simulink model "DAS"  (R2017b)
settings: Solver=FixedStepDiscrete  StartTime=0.0  StopTime=10.0  FixedStep=0.01  RelTol=1e-3  EnableMultiTasking=on
undefined symbols (not defined in the file): CcDAS_ACModeCurtLim_A, CcDAS_ACModeCurtTiLim_ms, CcDAS_BMSOperationConfirmTi_ms, CcDAS_CellMaxTempLim1_C, CcDAS_CellMaxTempLim2_C, CcDAS_CellMaxTempLim3_C, CcDAS_CellMaxTempLim4_C, CcDAS_CellMinTempHiLim_C, CcDAS_CellMinTempLowLim_C, CcDAS_CellMinTempMidLim_C, CcDAS_CellTempDiffLim_C, CcDAS_DCModeCurtTiLim_ms, CcDAS_HVSafetyNVMStoreTi_ms, CcDAS_OCVSOCDiffLim1_numb, CcDAS_OCVSOCDiffLim2_numb, CcDAS_PackCurrLim_A, CcDAS_SOCHighLim_numb, CcDAS_SOCLowerLim_numb, CcDAS_SOHLowerLim_numb, CcDAS_SOHLowerLimSale_numb, DAS_MIN2MS_NUMB, DAS_RUNTIME100_MS, DAS_RUNTIME10_MS, DAS_STATSTIMEMAX_MIN, DAS_STATSTIMEMIN_MIN, DAS_STATSTIMESMAX_NUMB, DAS_STATSTIMESMIN_NUMB, DAS_TIMESONE_NUMB, Enum_CTCCtrCtlConnMode
libraries: AIWAYS_Powertrain_BMS_lib x268
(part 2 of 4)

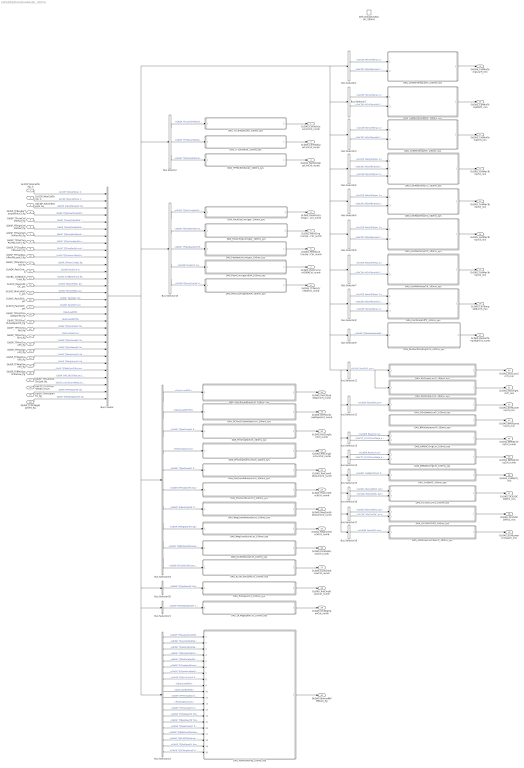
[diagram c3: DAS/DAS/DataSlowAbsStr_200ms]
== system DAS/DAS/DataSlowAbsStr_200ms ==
  GcCDP_MinCellTemp_C : Inport
  GcCDP_MaxCellTemp_C : Inport  Port=2
  GbCDP_AllCellTempVld_flg : Inport  Port=3
  GbISP_TFBusbarTempHiFltLv3_flg : Inport  Port=4
  GbISP_TFLowCellVoltSaf_flg : Inport  Port=5
  GbISP_TFHighCellVoltSaf_flg : Inport  Port=6
  GbISP_TFPackVoltHiAlrmFlt_flg : Inport  Port=7
  GbISP_TFDisChrgPwrFltLevel3_flg : Inport  Port=8
  GbISP_TFChrgPwrFltLevel3_flg : Inport  Port=9
  GbISP_TFFeedbackPwrFltLevel3_flg : Inport  Port=10
  GbISP_TFPackCrntSaf_flg : Inport  Port=11
  GcHDP_PackCrnt_A : Inport  Port=12
  GaCBC_CellBalCtlCmd_flg : Inport  Port=13
  GcSOC_MaxCellSOC_pct : Inport  Port=14
  GcSOC_MinCellSOC_pct : Inport  Port=15
  GcSOC_PackSOC_pct : Inport  Port=16
  GcSOH_PackSOH_pct : Inport  Port=17
  GbISP_TFPosCtlLoadOpenFlt_flg : Inport  Port=18
  GbISP_TFDCPosCtlLoadOpenFlt_flg : Inport  Port=19
  GbISP_TFPreChrgFail_flg : Inport  Port=20
  GbISP_TFPreChrgShrt_flg : Inport  Port=21
  GbISP_TFPosCloseFlt_flg : Inport  Port=22
  GbISP_TFPosOpenFlt_flg : Inport  Port=23
  GbISP_TFNegCloseFlt_flg : Inport  Port=24
  GbISP_TFNegOpenFlt_flg : Inport  Port=25
  GbISP_TFBMUSpyStTooLow_flg : Inport  Port=26
  GbISP_TFKL30CStTooLow_flg : Inport  Port=27
  GeCTC_CtrCtlConnMode_enum : Inport  Port=28
  GbISP_TFPreOpenFlt_flg : Inport  Port=29
  GbISP_TFDCNegOpenFlt_flg : Inport  Port=30
  DAS_DataSlowAbsStr_200ms : TriggerPort  TriggerType=function-call  VariantControl=(inherit)
  Bus Creator : BusCreator  Inputs=30
  Bus Selector : BusSelector  OutputSignals=GbISP_TFLowCellVoltSaf_flg,GbISP_TFHighCellVoltSaf_flg,GbISP_TFPackVoltHiAlrmFlt_flg
  Bus Selector1 : BusSelector  OutputSignals=GcCDP_MinCellTemp_C,GbCDP_AllCellTempVld_flg
  Bus Selector10 : BusSelector  OutputSignals=GbISP_TFDisChrgPwrFltLevel3_flg,GbISP_TFChrgPwrFltLevel3_flg,GbISP_TFFeedbackPwrFltLevel3_flg,GcHDP_PackCrnt_A,GbISP_TFPackCrntSaf_flg
  Bus Selector11 : BusSelector  OutputSignals=GcSOC_PackSOC_pct
  Bus Selector12 : BusSelector  OutputSignals=GcSOH_PackSOH_pct
  Bus Selector13 : BusSelector  OutputSignals=GcHDP_PackCrnt_A,GeCTC_CtrCtlConnMode_enum
  Bus Selector14 : BusSelector  OutputSignals=GcHDP_PackCrnt_A,GeCTC_CtrCtlConnMode_enum
  Bus Selector15 : BusSelector  OutputSignals=GaCBC_CellBalCtlCmd_flg
  Bus Selector16 : BusSelector  OutputSignals=GcSOC_MaxCellSOC_pct,GcSOC_MinCellSOC_pct
  Bus Selector17 : BusSelector  OutputSignals=GcSOC_MaxCellSOC_pct,GcSOC_MinCellSOC_pct
  Bus Selector18 : BusSelector  OutputSignals=OpenLoadPOS,OpenLoadDCPOS,GbISP_TFPreChrgFail_flg,PreChrgOverCurt,GbISP_TFPosCloseFlt_flg,GbISP_TFPosOpenFlt_flg,GbISP_TFNegCloseFlt_flg,GbISP_TFNegOpenFlt_flg,GbISP_TFBMUSpyStTooLow_flg,GbISP_TFKL30CStTooLow_flg
  Bus Selector19 : BusSelector  OutputSignals=GcSOH_PackSOH_pct
  Bus Selector2 : BusSelector  OutputSignals=GcCDP_MinCellTemp_C,GbCDP_AllCellTempVld_flg
  Bus Selector20 : BusSelector  OutputSignals=GbISP_TFPreOpenFlt_flg
  Bus Selector21 : BusSelector  OutputSignals=GbISP_TFDCNegOpenFlt_flg
  Bus Selector22 : BusSelector  OutputSignals=GbISP_TFBusbarTempHiFltLv3_flg,GbISP_TFLowCellVoltSaf_flg,GbISP_TFHighCellVoltSaf_flg,GbISP_TFPackVoltHiAlrmFlt_flg,GbISP_TFDisChrgPwrFltLevel3_flg,GbISP_TFChrgPwrFltLevel3_flg,GbISP_TFFeedbackPwrFltLevel3_flg,GbISP_TFPackCrntSaf_flg,OpenLoadPOS,OpenLoadDCPOS,GbISP_TFPreChrgFail_flg,PreChrgOverCurt,GbISP_TFPosCloseFlt_flg,GbISP_TFPosOpenFlt_flg,GbISP_TFNegOpenFlt_flg,GbISP_TFNegCloseFlt_flg,GbISP_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
  Bus Selector3 : BusSelector  OutputSignals=GcCDP_MinCellTemp_C,GbCDP_AllCellTempVld_flg
  Bus Selector4 : BusSelector  OutputSignals=GcCDP_MaxCellTemp_C,GbCDP_AllCellTempVld_flg,GcCDP_MinCellTemp_C
  Bus Selector5 : BusSelector  OutputSignals=GcCDP_MaxCellTemp_C,GbCDP_AllCellTempVld_flg
  Bus Selector6 : BusSelector  OutputSignals=GcCDP_MaxCellTemp_C,GbCDP_AllCellTempVld_flg
  Bus Selector7 : BusSelector  OutputSignals=GcCDP_MaxCellTemp_C,GbCDP_AllCellTempVld_flg
  Bus Selector8 : BusSelector  OutputSignals=GcCDP_MaxCellTemp_C,GbCDP_AllCellTempVld_flg,GcCDP_MinCellTemp_C
  Bus Selector9 : BusSelector  OutputSignals=GbISP_TFBusbarTempHiFltLv3_flg
  DAS_BMSACChrgCnt_100ms_sys : Subsystem  TreatAsAtomicUnit=on
  DAS_BMSDCChrgCnt_100ms_sys : Subsystem  TreatAsAtomicUnit=on
  DAS_BMSOperationTi_100ms_sys : Subsystem  TreatAsAtomicUnit=on
  DAS_BusbarTempHighCnt_100ms_sys : Subsystem  TreatAsAtomicUnit=on
  DAS_CellBalTi_100ms_sys : Subsystem  TreatAsAtomicUnit=on
  DAS_CellMaxTempTi1_100ms_sys : Subsystem  TreatAsAtomicUnit=on
  DAS_CellMaxTempTi2_100ms_sys : Subsystem  TreatAsAtomicUnit=on
  DAS_CellMaxTempTi3_100ms_sys : Subsystem  TreatAsAtomicUnit=on
  DAS_CellMaxTempTi4_100ms_sys : Subsystem  TreatAsAtomicUnit=on
  DAS_CellMinTempHiTi_100ms_sys : Subsystem  TreatAsAtomicUnit=on
  DAS_CellMinTempLowTi_100ms_sys : Subsystem  TreatAsAtomicUnit=on
  DAS_CellMinTempMidTi_100ms_sys : Subsystem  TreatAsAtomicUnit=on
  DAS_CellTempDiffTi_100ms_sys : Subsystem  TreatAsAtomicUnit=on
  DAS_DCNegOpenCnt_100ms_sys : Subsystem  TreatAsAtomicUnit=on
  DAS_DCPosCtlLoadOpenCnt_100ms_sys : Subsystem  TreatAsAtomicUnit=on
  DAS_FeedbackCurrUppr_100ms_sys : Subsystem  TreatAsAtomicUnit=on
  DAS_KL30CVoltLowCnt_100ms_sys : Subsystem  TreatAsAtomicUnit=on
  DAS_KL30VoltLowCnt_100ms_sys : Subsystem  TreatAsAtomicUnit=on
  DAS_NVMStoreFlg_100ms_sys : Subsystem  TreatAsAtomicUnit=on
  DAS_NegContAdhesionCnt_100ms_sys : Subsystem  TreatAsAtomicUnit=on
  DAS_NegContStuckCnt_100ms_sys : Subsystem  TreatAsAtomicUnit=on
  DAS_OCVSOCDiff1_100ms_sys : Subsystem  TreatAsAtomicUnit=on
  DAS_OCVSOCDiff2_100ms_sys : Subsystem  TreatAsAtomicUnit=on
  DAS_PACKCurrUppr600A_100ms_sys : Subsystem  TreatAsAtomicUnit=on
  DAS_PackChrgCurrUppr_100ms_sys : Subsystem  TreatAsAtomicUnit=on
  DAS_PackCurrUppr500A_100ms_sys : Subsystem  TreatAsAtomicUnit=on
  DAS_PackDisCurrUppr_100ms_sys : Subsystem  TreatAsAtomicUnit=on
  DAS_PosContAdhesionCnt_100ms_sys : Subsystem  TreatAsAtomicUnit=on
  DAS_PosContStuckCnt_100ms_sys : Subsystem  TreatAsAtomicUnit=on
  DAS_PosCtlLoadOpenCnt_100ms_sys : Subsystem  TreatAsAtomicUnit=on
  DAS_PreChrgFailCnt_100ms_sys : Subsystem  TreatAsAtomicUnit=on
  DAS_PreChrgOverCurtCnt_100ms_sys : Subsystem  TreatAsAtomicUnit=on
  DAS_PreOpenCnt_100ms_sys : Subsystem  TreatAsAtomicUnit=on
  DAS_SOCHighLimTi_100ms_sys : Subsystem  TreatAsAtomicUnit=on
  DAS_SOCUpprLimTi_100ms_sys : Subsystem  TreatAsAtomicUnit=on
  DAS_SOHLowerLimSaleTi_100ms_sys : Subsystem  TreatAsAtomicUnit=on
  DAS_SOHLowerLimTi_100ms_sys : Subsystem  TreatAsAtomicUnit=on
  DAS_TFCellVoltHi_100ms_sys : Subsystem  TreatAsAtomicUnit=on
  DAS_TFCellVoltLowr_100ms_sys : Subsystem  TreatAsAtomicUnit=on
  DAS_TFPACKVoltLowr_100ms_sys : Subsystem  TreatAsAtomicUnit=on
  GcDAS_CellVoltLowrLimCnt_numb : Outport
  GcDAS_CellVoltUpprLimCnt_numb : Outport  Port=2
  GcDAS_BattVoltUpprLimCnt_numb : Outport  Port=3
  GcDAS_PackDisCurrUpprLimCnt_numb : Outport  Port=4
  GcDAS_PackChrgCurrUpprLimCnt_numb : Outport  Port=5
  GcDAS_FeedbackCurrUpprLimCnt_numb : Outport  Port=6
  GcDAS_PackCurrLim500ACnt_numb : Outport  Port=7
  GcDAS_TFPackCrntSafCnt_numb : Outport  Port=8
  GcDAS_CellMinTempLowTi_min : Outport  Port=9
  GcDAS_CellMinTempMidTi_min : Outport  Port=10
  GcDAS_CellMinTempHiTi_min : Outport  Port=11
  GcDAS_CellMaxTempTi1_min : Outport  Port=12
  GcDAS_CellMaxTempTi2_min : Outport  Port=13
  GcDAS_CellMaxTempTi3_min : Outport  Port=14
  GcDAS_CellMaxTempTi4_min : Outport  Port=15
  GcDAS_CellTempDiffLimTi_min : Outport  Port=16
  GcDAS_BusbarTempHighCnt_numb : Outport  Port=17
  GcDAS_PosCtlLoadOpenCnt_numb : Outport  Port=18
  GcDAS_DCPosCtlLoadOpenCnt_numb : Outport  Port=19
  GcDAS_PreChrgFailCnt_numb : Outport  Port=20
  GcDAS_PreChrgOvrCurrCnt_numb : Outport  Port=21
  GcDAS_PosContAdhesionCnt_numb : Outport  Port=22
  GcDAS_PosContStuckCnt_numb : Outport  Port=23
  GcDAS_NegContAdhesionCnt_numb : Outport  Port=24
  GcDAS_NegContStuckCnt_numb : Outport  Port=25
  GcDAS_KL30VoltLowCnt_numb : Outport  Port=26
  GcDAS_KL30CVoltLowCnt_numb : Outport  Port=27
  GcDAS_PreChrgOpenCnt_numb : Outport  Port=28
  GcDAS_DCNegOpenCnt_numb : Outport  Port=29
  GcDAS_SOCLowLimTi_min : Outport  Port=30
  GcDAS_SOCHighLimTi_min : Outport  Port=31
  GcDAS_SOHLowerLimTi_min : Outport  Port=32
  GcDAS_BMSOperationTi_min : Outport  Port=33
  GcDAS_BMSACChrgCnt_numb : Outport  Port=34
  GcDAS_BMSDCChrgCnt_numb : Outport  Port=35
  GcDAS_CellBalTi_min : Outport  Port=36
  GcDAS_OCVSOCDiffTi1_min : Outport  Port=37
  GcDAS_OCVSOCDiffTi2_min : Outport  Port=38
  GcDAS_SOHLowerLimSaleTi_min : Outport  Port=39
  GbDAS_NormalNVMStore_flg : Outport  Port=40
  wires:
  GcCDP_MinCellTemp_C/1 -> Bus Creator/1  "GcCDP_MinCellTemp_C"
  GcCDP_MaxCellTemp_C/1 -> Bus Creator/2  "GcCDP_MaxCellTemp_C"
  GbCDP_AllCellTempVld_flg/1 -> Bus Creator/3  "GbCDP_AllCellTempVld_flg"
  GbISP_TFBusbarTempHiFltLv3_flg/1 -> Bus Creator/4  "GbISP_TFBusbarTempHiFltLv3_flg"
  GbISP_TFLowCellVoltSaf_flg/1 -> Bus Creator/5  "GbISP_TFLowCellVoltSaf_flg"
  GbISP_TFHighCellVoltSaf_flg/1 -> Bus Creator/6  "GbISP_TFHighCellVoltSaf_flg"
  GbISP_TFPackVoltHiAlrmFlt_flg/1 -> Bus Creator/7  "GbISP_TFPackVoltHiAlrmFlt_flg"
  GbISP_TFDisChrgPwrFltLevel3_flg/1 -> Bus Creator/8  "GbISP_TFDisChrgPwrFltLevel3_flg"
  GbISP_TFChrgPwrFltLevel3_flg/1 -> Bus Creator/9  "GbISP_TFChrgPwrFltLevel3_flg"
  GbISP_TFFeedbackPwrFltLevel3_flg/1 -> Bus Creator/10  "GbISP_TFFeedbackPwrFltLevel3_flg"
  GbISP_TFPackCrntSaf_flg/1 -> Bus Creator/11  "GbISP_TFPackCrntSaf_flg"
  GcHDP_PackCrnt_A/1 -> Bus Creator/12  "GcHDP_PackCrnt_A"
  GaCBC_CellBalCtlCmd_flg/1 -> Bus Creator/13  "GaCBC_CellBalCtlCmd_flg"
  GcSOC_MaxCellSOC_pct/1 -> Bus Creator/14  "GcSOC_MaxCellSOC_pct"
  GcSOC_MinCellSOC_pct/1 -> Bus Creator/15  "GcSOC_MinCellSOC_pct"
  GcSOC_PackSOC_pct/1 -> Bus Creator/16  "GcSOC_PackSOC_pct"
  GcSOH_PackSOH_pct/1 -> Bus Creator/17  "GcSOH_PackSOH_pct"
  GbISP_TFPosCtlLoadOpenFlt_flg/1 -> Bus Creator/18  "OpenLoadPOS"
  GbISP_TFDCPosCtlLoadOpenFlt_flg/1 -> Bus Creator/19  "OpenLoadDCPOS"
  GbISP_TFPreChrgFail_flg/1 -> Bus Creator/20  "GbISP_TFPreChrgFail_flg"
  GbISP_TFPreChrgShrt_flg/1 -> Bus Creator/21  "PreChrgOverCurt"
  GbISP_TFPosCloseFlt_flg/1 -> Bus Creator/22  "GbISP_TFPosCloseFlt_flg"
  GbISP_TFPosOpenFlt_flg/1 -> Bus Creator/23  "GbISP_TFPosOpenFlt_flg"
  GbISP_TFNegCloseFlt_flg/1 -> Bus Creator/24  "GbISP_TFNegCloseFlt_flg"
  GbISP_TFNegOpenFlt_flg/1 -> Bus Creator/25  "GbISP_TFNegOpenFlt_flg"
  GbISP_TFBMUSpyStTooLow_flg/1 -> Bus Creator/26  "GbISP_TFBMUSpyStTooLow_flg"
  GbISP_TFKL30CStTooLow_flg/1 -> Bus Creator/27  "GbISP_TFKL30CStTooLow_flg"
  GeCTC_CtrCtlConnMode_enum/1 -> Bus Creator/28  "GeCTC_CtrCtlConnMode_enum"
  Bus Selector/1 -> DAS_TFCellVoltLowr_100ms_sys/1(GbISP_TFLowCellVoltSaf_flg)  "<GbISP_TFLowCellVoltSaf_flg>"
  Bus Selector/2 -> DAS_TFCellVoltHi_100ms_sys/1(GbISP_TFHighCellVoltSaf_flg)  "<GbISP_TFHighCellVoltSaf_flg>"
  Bus Selector/3 -> DAS_TFPACKVoltLowr_100ms_sys/1(GbISP_TFPackVoltHiAlrmFlt_flg)  "<GbISP_TFPackVoltHiAlrmFlt_flg>"
  Bus Selector1/1 -> DAS_CellMinTempLowTi_100ms_sys/1(GcCDP_MinCellTemp_C)  "<GcCDP_MinCellTemp_C>"
  Bus Selector1/2 -> DAS_CellMinTempLowTi_100ms_sys/2(GbCDP_AllCellTempVld_flg)  "<GbCDP_AllCellTempVld_flg>"
  Bus Selector2/1 -> DAS_CellMinTempMidTi_100ms_sys/1(GcCDP_MinCellTemp_C)  "<GcCDP_MinCellTemp_C>"
  Bus Selector2/2 -> DAS_CellMinTempMidTi_100ms_sys/2(GbCDP_AllCellTempVld_flg)  "<GbCDP_AllCellTempVld_flg>"
  Bus Selector3/1 -> DAS_CellMinTempHiTi_100ms_sys/1(GcCDP_MinCellTemp_C)  "<GcCDP_MinCellTemp_C>"
  Bus Selector3/2 -> DAS_CellMinTempHiTi_100ms_sys/2(GbCDP_AllCellTempVld_flg)  "<GbCDP_AllCellTempVld_flg>"
  Bus Selector4/1 -> DAS_CellMaxTempTi1_100ms_sys/1(GcCDP_MaxCellTemp_C)  "<GcCDP_MaxCellTemp_C>"
  Bus Selector4/2 -> DAS_CellMaxTempTi1_100ms_sys/2(GbCDP_AllCellTempVld_flg)  "<GbCDP_AllCellTempVld_flg>"
  Bus Selector4/3 -> DAS_CellMaxTempTi1_100ms_sys/3(GcCDP_MinCellTemp_C)  "<GcCDP_MinCellTemp_C>"
  Bus Selector5/1 -> DAS_CellMaxTempTi2_100ms_sys/1(GcCDP_MaxCellTemp_C)  "<GcCDP_MaxCellTemp_C>"
  Bus Selector5/2 -> DAS_CellMaxTempTi2_100ms_sys/2(GbCDP_AllCellTempVld_flg)  "<GbCDP_AllCellTempVld_flg>"
  Bus Selector6/1 -> DAS_CellMaxTempTi3_100ms_sys/1(GcCDP_MaxCellTemp_C)  "<GcCDP_MaxCellTemp_C>"
  Bus Selector6/2 -> DAS_CellMaxTempTi3_100ms_sys/2(GbCDP_AllCellTempVld_flg)  "<GbCDP_AllCellTempVld_flg>"
  Bus Selector7/1 -> DAS_CellMaxTempTi4_100ms_sys/1(GcCDP_MaxCellTemp_C)  "<GcCDP_MaxCellTemp_C>"
  Bus Selector7/2 -> DAS_CellMaxTempTi4_100ms_sys/2(GbCDP_AllCellTempVld_flg)  "<GbCDP_AllCellTempVld_flg>"
  Bus Selector8/1 -> DAS_CellTempDiffTi_100ms_sys/1(GcCDP_MaxCellTemp_C)  "<GcCDP_MaxCellTemp_C>"
  Bus Selector8/2 -> DAS_CellTempDiffTi_100ms_sys/2(GbCDP_AllCellTempVld_flg)  "<GbCDP_AllCellTempVld_flg>"
  Bus Selector8/3 -> DAS_CellTempDiffTi_100ms_sys/3(GcCDP_MinCellTemp_C)  "<GcCDP_MinCellTemp_C>"
  Bus Selector9/1 -> DAS_BusbarTempHighCnt_100ms_sys/1(GbISP_TFBusbarTempHiFltLv3_flg)  "<GbISP_TFBusbarTempHiFltLv3_flg>"
  Bus Selector10/1 -> DAS_PackDisCurrUppr_100ms_sys/1(GbISP_TFDisChrgPwrFltLevel3_flg)  "<GbISP_TFDisChrgPwrFltLevel3_flg>"
  Bus Selector10/2 -> DAS_PackChrgCurrUppr_100ms_sys/1(GbISP_TFChrgPwrFltLevel3_flg)  "<GbISP_TFChrgPwrFltLevel3_flg>"
  Bus Selector10/3 -> DAS_FeedbackCurrUppr_100ms_sys/1(GbISP_TFFeedbackPwrFltLevel3_flg)  "<GbISP_TFFeedbackPwrFltLevel3_flg>"
  Bus Selector10/4 -> DAS_PackCurrUppr500A_100ms_sys/1(GcHDP_PackCrnt_A)  "<GcHDP_PackCrnt_A>"
  Bus Selector10/5 -> DAS_PACKCurrUppr600A_100ms_sys/1(GbISP_TFPackCrntSaf_flg)  "<GbISP_TFPackCrntSaf_flg>"
  Bus Selector11/1 -> DAS_SOCHighLimTi_100ms_sys/1(GcSOC_PackSOC_pct), DAS_SOCUpprLimTi_100ms_sys/1(GcSOC_PackSOC_pct)  "<GcSOC_PackSOC_pct>"
  Bus Selector12/1 -> DAS_SOHLowerLimTi_100ms_sys/1(GcSOH_PackSOH_pct)  "<GcSOH_PackSOH_pct>"
  Bus Selector13/1 -> DAS_BMSACChrgCnt_100ms_sys/1(GcHDP_PackCrnt_A)  "<GcHDP_PackCrnt_A>"
  Bus Selector13/2 -> DAS_BMSACChrgCnt_100ms_sys/2(GeCTC_CtrCtlConnMode_enum)  "<GeCTC_CtrCtlConnMode_enum>"
  Bus Selector14/1 -> DAS_BMSDCChrgCnt_100ms_sys/1(GcHDP_PackCrnt_A)  "<GcHDP_PackCrnt_A>"
  Bus Selector14/2 -> DAS_BMSDCChrgCnt_100ms_sys/2(GeCTC_CtrCtlConnMode_enum)  "<GeCTC_CtrCtlConnMode_enum>"
  Bus Selector15/1 -> DAS_CellBalTi_100ms_sys/1(GaCBC_CellBalCtlCmd_flg)  "<GaCBC_CellBalCtlCmd_flg>"
  Bus Selector16/1 -> DAS_OCVSOCDiff1_100ms_sys/1(GcSOC_MaxCellSOC_pct)  "<GcSOC_MaxCellSOC_pct>"
  Bus Selector16/2 -> DAS_OCVSOCDiff1_100ms_sys/2(GcSOC_MinCellSOC_pct)  "<GcSOC_MinCellSOC_pct>"
  Bus Selector17/1 -> DAS_OCVSOCDiff2_100ms_sys/1(GcSOC_MaxCellSOC_pct)  "<GcSOC_MaxCellSOC_pct>"
  Bus Selector17/2 -> DAS_OCVSOCDiff2_100ms_sys/2(GcSOC_MinCellSOC_pct)  "<GcSOC_MinCellSOC_pct>"
  Bus Selector18/1 -> DAS_PosCtlLoadOpenCnt_100ms_sys/1(GcISP_ShutDownPosCtlLoadOpen_flg)  "<OpenLoadPOS>"
  Bus Selector18/2 -> DAS_DCPosCtlLoadOpenCnt_100ms_sys/1(GcISP_ShutDownDCPosChrgCtlLoadOpen_flg)  "<OpenLoadDCPOS>"
  Bus Selector18/3 -> DAS_PreChrgFailCnt_100ms_sys/1(GbISP_TFPreChrgFail_flg)  "<GbISP_TFPreChrgFail_flg>"
  Bus Selector18/4 -> DAS_PreChrgOverCurtCnt_100ms_sys/1(GbISP_TFPreChrgOverCurt_flg)  "<PreChrgOverCurt>"
  Bus Selector18/5 -> DAS_PosContAdhesionCnt_100ms_sys/1(GbISP_TFPosCloseFlt_flg)  "<GbISP_TFPosCloseFlt_flg>"
  Bus Selector18/6 -> DAS_PosContStuckCnt_100ms_sys/1(GbISP_TFPosOpenFlt_flg)  "<GbISP_TFPosOpenFlt_flg>"
  Bus Selector18/7 -> DAS_NegContAdhesionCnt_100ms_sys/1(GbISP_TFNegCloseFlt_flg)  "<GbISP_TFNegCloseFlt_flg>"
  Bus Selector18/8 -> DAS_NegContStuckCnt_100ms_sys/1(GbISP_TFNegOpenFlt_flg)  "<GbISP_TFNegOpenFlt_flg>"
  Bus Selector18/9 -> DAS_KL30VoltLowCnt_100ms_sys/1(GbISP_TFBMUSpyStTooLow_flg)  "<GbISP_TFBMUSpyStTooLow_flg>"
  Bus Selector18/10 -> DAS_KL30CVoltLowCnt_100ms_sys/1(GbISP_TFKL30CStTooLow_flg)  "<GbISP_TFKL30CStTooLow_flg>"
  DAS_TFCellVoltLowr_100ms_sys/1(GcDAS_CellVoltLowrLimCnt_numb) -> GcDAS_CellVoltLowrLimCnt_numb/1
  DAS_TFCellVoltHi_100ms_sys/1(GcDAS_CellVoltUpprLimCnt_numb) -> GcDAS_CellVoltUpprLimCnt_numb/1
  DAS_TFPACKVoltLowr_100ms_sys/1(GcDAS_BattVoltUpprLimCnt_numb) -> GcDAS_BattVoltUpprLimCnt_numb/1
  DAS_PackDisCurrUppr_100ms_sys/1(GcDAS_PackDisCurrUpprLimCnt_numb) -> GcDAS_PackDisCurrUpprLimCnt_numb/1
  DAS_PackChrgCurrUppr_100ms_sys/1(GcDAS_PackChrgCurrUpprLimCnt_numb) -> GcDAS_PackChrgCurrUpprLimCnt_numb/1
  DAS_FeedbackCurrUppr_100ms_sys/1(GcDAS_FeedbackCurrUpprLimCnt_numb) -> GcDAS_FeedbackCurrUpprLimCnt_numb/1
  DAS_PackCurrUppr500A_100ms_sys/1(GcDAS_PackCurrLim500ACnt_numb) -> GcDAS_PackCurrLim500ACnt_numb/1
  DAS_PACKCurrUppr600A_100ms_sys/1(GcDAS_TFPackCrntSafCnt_numb) -> GcDAS_TFPackCrntSafCnt_numb/1
  DAS_CellMinTempLowTi_100ms_sys/1(GcDAS_CellMinTempLowTi_min) -> GcDAS_CellMinTempLowTi_min/1
  DAS_CellMinTempMidTi_100ms_sys/1(GcDAS_CellMinTempMidTi_min) -> GcDAS_CellMinTempMidTi_min/1
  DAS_CellMinTempHiTi_100ms_sys/1(GcDAS_CellMinTempHiTi_min) -> GcDAS_CellMinTempHiTi_min/1
  DAS_CellMaxTempTi1_100ms_sys/1(GcDAS_CellMaxTempTi1_min) -> GcDAS_CellMaxTempTi1_min/1
  DAS_CellMaxTempTi2_100ms_sys/1(GcDAS_CellMaxTempTi2_min) -> GcDAS_CellMaxTempTi2_min/1
  DAS_CellMaxTempTi3_100ms_sys/1(GcDAS_CellMaxTempTi3_min) -> GcDAS_CellMaxTempTi3_min/1
  DAS_CellMaxTempTi4_100ms_sys/1(GcDAS_CellMaxTempTi4_min) -> GcDAS_CellMaxTempTi4_min/1
  DAS_CellTempDiffTi_100ms_sys/1(GcDAS_CellTempDiffLimTi_min) -> GcDAS_CellTempDiffLimTi_min/1
  DAS_BusbarTempHighCnt_100ms_sys/1(GcDAS_BusbarTempHighCnt_numb) -> GcDAS_BusbarTempHighCnt_numb/1
  Bus Selector19/1 -> DAS_SOHLowerLimSaleTi_100ms_sys/1(GcSOH_PackSOH_pct)  "<GcSOH_PackSOH_pct>"
  GbISP_TFPreOpenFlt_flg/1 -> Bus Creator/29  "GbISP_TFPreOpenFlt_flg"
  GbISP_TFDCNegOpenFlt_flg/1 -> Bus Creator/30  "GbISP_TFDCNegOpenFlt_flg"
  Bus Selector20/1 -> DAS_PreOpenCnt_100ms_sys/1(GbISP_TFPreOpenFlt_flg)  "<GbISP_TFPreOpenFlt_flg>"
  Bus Selector21/1 -> DAS_DCNegOpenCnt_100ms_sys/1(GbISP_TFDCNegOpenFlt_flg)  "<GbISP_TFDCNegOpenFlt_flg>"
  DAS_PosCtlLoadOpenCnt_100ms_sys/1(GcDAS_PosCtlLoadOpenCnt_numb) -> GcDAS_PosCtlLoadOpenCnt_numb/1
  DAS_DCPosCtlLoadOpenCnt_100ms_sys/1(GcDAS_DCPosCtlLoadOpenCnt_numb) -> GcDAS_DCPosCtlLoadOpenCnt_numb/1
  DAS_PreChrgFailCnt_100ms_sys/1(GcDAS_PreChrgFailCnt_numb) -> GcDAS_PreChrgFailCnt_numb/1
  DAS_PreChrgOverCurtCnt_100ms_sys/1(GcDAS_PreChrgOvrCurrCnt_numb) -> GcDAS_PreChrgOvrCurrCnt_numb/1
  DAS_PosContAdhesionCnt_100ms_sys/1(GcDAS_PosContAdhesionCnt_numb) -> GcDAS_PosContAdhesionCnt_numb/1
  DAS_PosContStuckCnt_100ms_sys/1(GcDAS_PosContStuckCnt_numb) -> GcDAS_PosContStuckCnt_numb/1
  DAS_NegContAdhesionCnt_100ms_sys/1(GcDAS_NegContAdhesionCnt_numb) -> GcDAS_NegContAdhesionCnt_numb/1
  DAS_NegContStuckCnt_100ms_sys/1(GcDAS_NegContStuckCnt_numb) -> GcDAS_NegContStuckCnt_numb/1
  DAS_KL30VoltLowCnt_100ms_sys/1(GcDAS_KL30VoltLowCnt_numb) -> GcDAS_KL30VoltLowCnt_numb/1
  DAS_KL30CVoltLowCnt_100ms_sys/1(GcDAS_KL30CVoltLowCnt_numb) -> GcDAS_KL30CVoltLowCnt_numb/1
  DAS_PreOpenCnt_100ms_sys/1(GcDAS_PreChrgOpenCnt_numb) -> GcDAS_PreChrgOpenCnt_numb/1
  DAS_DCNegOpenCnt_100ms_sys/1(GcDAS_DCNegOpenCnt_numb) -> GcDAS_DCNegOpenCnt_numb/1
  DAS_SOCUpprLimTi_100ms_sys/1(GcDAS_SOCLowLimTi_min) -> GcDAS_SOCLowLimTi_min/1
  DAS_SOCHighLimTi_100ms_sys/1(GcDAS_SOCHighLimTi_min) -> GcDAS_SOCHighLimTi_min/1
  DAS_SOHLowerLimTi_100ms_sys/1(GcDAS_SOHLowerLimTi_min) -> GcDAS_SOHLowerLimTi_min/1
  DAS_BMSOperationTi_100ms_sys/1(GcDAS_BMSOperationTi_min) -> GcDAS_BMSOperationTi_min/1
  DAS_BMSACChrgCnt_100ms_sys/1(GcDAS_BMSACChrgCnt_numb) -> GcDAS_BMSACChrgCnt_numb/1
  DAS_BMSDCChrgCnt_100ms_sys/1(GcDAS_BMSDCChrgCnt_numb) -> GcDAS_BMSDCChrgCnt_numb/1
  DAS_CellBalTi_100ms_sys/1(GcDAS_CellBalTi_min) -> GcDAS_CellBalTi_min/1
  DAS_OCVSOCDiff1_100ms_sys/1(GcDAS_OCVSOCDiffTi1_min) -> GcDAS_OCVSOCDiffTi1_min/1
  DAS_OCVSOCDiff2_100ms_sys/1(GcDAS_OCVSOCDiffTi2_min) -> GcDAS_OCVSOCDiffTi2_min/1
  DAS_SOHLowerLimSaleTi_100ms_sys/1(GcDAS_SOHLowerLimSaleTi_min) -> GcDAS_SOHLowerLimSaleTi_min/1
  Bus Creator/1 -> Bus Selector22/1, Bus Selector21/1, Bus Selector20/1, Bus Selector18/1, Bus Selector10/1, Bus Selector19/1, Bus Selector17/1, Bus Selector16/1, Bus Selector15/1, Bus Selector14/1, Bus Selector13/1, Bus Selector12/1, Bus Selector11/1, Bus Selector9/1, Bus Selector8/1, Bus Selector7/1, Bus Selector6/1, Bus Selector5/1, Bus Selector4/1, Bus Selector3/1, Bus Selector2/1, Bus Selector1/1, Bus Selector/1
  Bus Selector22/1 -> DAS_NVMStoreFlg_100ms_sys/1(GbISP_TFBusbarTempHiFltLv3_flg)  "<GbISP_TFBusbarTempHiFltLv3_flg>"
  Bus Selector22/2 -> DAS_NVMStoreFlg_100ms_sys/2(GbISP_TFLowCellVoltSaf_flg)  "<GbISP_TFLowCellVoltSaf_flg>"
  Bus Selector22/3 -> DAS_NVMStoreFlg_100ms_sys/3(GbISP_TFHighCellVoltSaf_flg)  "<GbISP_TFHighCellVoltSaf_flg>"
  Bus Selector22/4 -> DAS_NVMStoreFlg_100ms_sys/4(GbISP_TFPackVoltHiAlrmFlt_flg)  "<GbISP_TFPackVoltHiAlrmFlt_flg>"
  Bus Selector22/5 -> DAS_NVMStoreFlg_100ms_sys/5(GbISP_TFDisChrgPwrFltLevel3_flg)  "<GbISP_TFDisChrgPwrFltLevel3_flg>"
  Bus Selector22/6 -> DAS_NVMStoreFlg_100ms_sys/6(GbISP_TFChrgPwrFltLevel3_flg)  "<GbISP_TFChrgPwrFltLevel3_flg>"
  Bus Selector22/7 -> DAS_NVMStoreFlg_100ms_sys/7(GbISP_TFFeedbackPwrFltLevel3_flg)  "<GbISP_TFFeedbackPwrFltLevel3_flg>"
  Bus Selector22/8 -> DAS_NVMStoreFlg_100ms_sys/8(GbISP_TFPackCrntSaf_flg)  "<GbISP_TFPackCrntSaf_flg>"
  Bus Selector22/9 -> DAS_NVMStoreFlg_100ms_sys/9(GbISP_TFPosCtlLoadOpenFlt_flg)  "<OpenLoadPOS>"
  Bus Selector22/10 -> DAS_NVMStoreFlg_100ms_sys/10(GbISP_TFDCPosCtlLoadOpenFlt_flg)  "<OpenLoadDCPOS>"
  Bus Selector22/11 -> DAS_NVMStoreFlg_100ms_sys/11(GbISP_TFPreChrgFail_flg)  "<GbISP_TFPreChrgFail_flg>"
  Bus Selector22/12 -> DAS_NVMStoreFlg_100ms_sys/12(GbISP_TFPreChrgShrt_flg)  "<PreChrgOverCurt>"
  Bus Selector22/13 -> DAS_NVMStoreFlg_100ms_sys/13(GbISP_TFPosCloseFlt_flg)  "<GbISP_TFPosCloseFlt_flg>"
  Bus Selector22/14 -> DAS_NVMStoreFlg_100ms_sys/14(GbISP_TFPosOpenFlt_flg)  "<GbISP_TFPosOpenFlt_flg>"
  Bus Selector22/15 -> DAS_NVMStoreFlg_100ms_sys/15(GbISP_TFNegCloseFlt_flg)  "<GbISP_TFNegOpenFlt_flg>"
  Bus Selector22/16 -> DAS_NVMStoreFlg_100ms_sys/16(GbISP_TFNegOpenFlt_flg)  "<GbISP_TFNegCloseFlt_flg>"
  Bus Selector22/17 -> DAS_NVMStoreFlg_100ms_sys/17(GbISP_TFBMUSpyStTooLow_flg)  "<GbISP_TFBMUSpyStTooLow_flg>"
  Bus Selector22/18 -> DAS_NVMStoreFlg_100ms_sys/18(GbISP_TFKL30CStTooLow_flg)  "<GbISP_TFKL30CStTooLow_flg>"
  Bus Selector22/19 -> DAS_NVMStoreFlg_100ms_sys/19(GbISP_TFPreOpenFlt_flg)  "<GbISP_TFPreOpenFlt_flg>"
  Bus Selector22/20 -> DAS_NVMStoreFlg_100ms_sys/20(GbISP_TFDCNegOpenFlt_flg)  "<GbISP_TFDCNegOpenFlt_flg>"
  DAS_NVMStoreFlg_100ms_sys/1(GbDAS_NormalNVMStore_flg) -> GbDAS_NormalNVMStore_flg/1

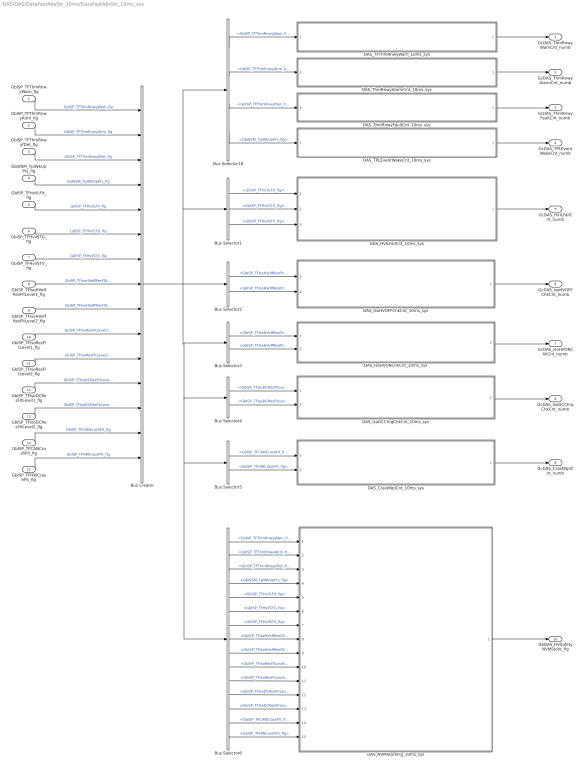
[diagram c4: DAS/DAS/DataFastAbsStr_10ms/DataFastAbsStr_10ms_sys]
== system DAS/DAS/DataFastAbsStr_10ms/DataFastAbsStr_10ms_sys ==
  GbISP_TFThmRnwyWarn_flg : Inport
  GbISP_TFThmRnwyAlrm_flg : Inport  Port=2
  GbISP_TFThmRnwyfDet_flg : Inport  Port=3
  GbWSM_TplWkUpPrs_flg : Inport  Port=4
  GbISP_TFHvilLFlt_flg : Inport  Port=5
  GbISP_TFHvilSTG_flg : Inport  Port=6
  GbISP_TFHvilSTV_flg : Inport  Port=7
  GbISP_TFIsoHVoffResFltLevel1_flg : Inport  Port=8
  GbISP_TFIsoHVoffResFltLevel2_flg : Inport  Port=9
  GbISP_TFIsoResFltLevel1_flg : Inport  Port=10
  GbISP_TFIsoResFltLevel2_flg : Inport  Port=11
  GbISP_TFIsoDCResFltLevel1_flg : Inport  Port=12
  GbISP_TFIsoDCResFltLevel2_flg : Inport  Port=13
  GbISP_TFCANCrashFlt_flg : Inport  Port=14
  GbISP_TFHWCrashFlt_flg : Inport  Port=15
  Bus Creator : BusCreator  Inputs=15
  Bus Selector1 : BusSelector  OutputSignals=GbISP_TFHvilLFlt_flg,GbISP_TFHvilSTG_flg,GbISP_TFHvilSTV_flg
  Bus Selector18 : BusSelector  OutputSignals=GbISP_TFThmRnwyWarn_flg,GbISP_TFThmRnwyAlrm_flg,GbISP_TFThmRnwyfDet_flg,GbWSM_TplWkUpPrs_flg
  Bus Selector2 : BusSelector  OutputSignals=GbISP_TFIsoHVoffResFltLevel1_flg,GbISP_TFIsoHVoffResFltLevel2_flg
  Bus Selector3 : BusSelector  OutputSignals=GbISP_TFIsoHVoffResFltLevel1_flg,GbISP_TFIsoHVoffResFltLevel2_flg
  Bus Selector4 : BusSelector  OutputSignals=GbISP_TFIsoDCResFltLevel1_flg,GbISP_TFIsoDCResFltLevel2_flg
  Bus Selector5 : BusSelector  OutputSignals=GbISP_TFCANCrashFlt_flg,GbISP_TFHWCrashFlt_flg
  Bus Selector6 : BusSelector  OutputSignals=GbISP_TFThmRnwyWarn_flg,GbISP_TFThmRnwyAlrm_flg,GbISP_TFThmRnwyfDet_flg,GbWSM_TplWkUpPrs_flg,GbISP_TFHvilLFlt_flg,GbISP_TFHvilSTG_flg,GbISP_TFHvilSTV_flg,GbISP_TFIsoHVoffResFltLevel1_flg,GbISP_TFIsoHVoffResFltLevel2_flg,GbISP_TFIsoResFltLevel1_flg,GbISP_TFIsoResFltLevel2_flg,GbISP_TFIsoDCResFltLevel1_flg,GbISP_TFIsoDCResFltLevel2_flg,GbISP_TFCANCrashFlt_flg,GbISP_TFHWCrashFlt_flg
  DAS_CrashNplCnt_10ms_sys : Subsystem  TreatAsAtomicUnit=on
  DAS_HVILFailCnt_10ms_sys : Subsystem  TreatAsAtomicUnit=on
  DAS_IsoDCChrgChkCnt_10ms_sys : Subsystem  TreatAsAtomicUnit=on
  DAS_IsoHVOFFChkCnt_10ms_sys : Subsystem  TreatAsAtomicUnit=on
  DAS_IsoHVONChkCnt_10ms_sys : Subsystem  TreatAsAtomicUnit=on
  DAS_NVMStoreFlg_10ms_sys : Subsystem  TreatAsAtomicUnit=on
  DAS_TFThmRnwyWarn_10ms_sys : Subsystem  TreatAsAtomicUnit=on
  DAS_TPLEventWakeCnt_10ms_sys : Subsystem  TreatAsAtomicUnit=on
  DAS_ThmRnwyAlarmCnt_10ms_sys : Subsystem  TreatAsAtomicUnit=on
  DAS_ThmRnwyFaultCnt_10ms_sys : Subsystem  TreatAsAtomicUnit=on
  GcDAS_ThmRnwyWarnCnt_numb : Outport
  GcDAS_ThmRnwyAlarmCnt_numb : Outport  Port=2
  GcDAS_ThmRnwyFaultCnt_numb : Outport  Port=3
  GcDAS_TPLEventWakeCnt_numb : Outport  Port=4
  GcDAS_HVILFailCnt_numb : Outport  Port=5
  GcDAS_IsoHVOFFChkCnt_numb : Outport  Port=6
  GcDAS_IsoHVONChkCnt_numb : Outport  Port=7
  GcDAS_IsoDCChrgChkCnt_numb : Outport  Port=8
  GcDAS_CrashNplCnt_numb : Outport  Port=9
  GbDAS_HVSafetyNVMStore_flg : Outport  Port=10
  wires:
  GbISP_TFHvilSTV_flg/1 -> Bus Creator/7  "GbISP_TFHvilSTV_flg"
  GbISP_TFHvilLFlt_flg/1 -> Bus Creator/5  "GbISP_TFHvilLFlt_flg"
  GbISP_TFIsoResFltLevel1_flg/1 -> Bus Creator/10  "GbISP_TFIsoResFltLevel1_flg"
  GbISP_TFIsoResFltLevel2_flg/1 -> Bus Creator/11  "GbISP_TFIsoResFltLevel2_flg"
  GbISP_TFIsoDCResFltLevel2_flg/1 -> Bus Creator/13  "GbISP_TFIsoDCResFltLevel2_flg"
  GbISP_TFIsoDCResFltLevel1_flg/1 -> Bus Creator/12  "GbISP_TFIsoDCResFltLevel1_flg"
  GbISP_TFHWCrashFlt_flg/1 -> Bus Creator/15  "GbISP_TFHWCrashFlt_flg"
  GbISP_TFCANCrashFlt_flg/1 -> Bus Creator/14  "GbISP_TFCANCrashFlt_flg"
  GbISP_TFThmRnwyWarn_flg/1 -> Bus Creator/1  "GbISP_TFThmRnwyWarn_flg"
  GbISP_TFThmRnwyAlrm_flg/1 -> Bus Creator/2  "GbISP_TFThmRnwyAlrm_flg"
  GbISP_TFThmRnwyfDet_flg/1 -> Bus Creator/3  "GbISP_TFThmRnwyfDet_flg"
  GbWSM_TplWkUpPrs_flg/1 -> Bus Creator/4  "GbWSM_TplWkUpPrs_flg"
  GbISP_TFHvilSTG_flg/1 -> Bus Creator/6  "GbISP_TFHvilSTG_flg"
  GbISP_TFIsoHVoffResFltLevel1_flg/1 -> Bus Creator/8  "GbISP_TFIsoHVoffResFltLevel1_flg"
  GbISP_TFIsoHVoffResFltLevel2_flg/1 -> Bus Creator/9  "GbISP_TFIsoHVoffResFltLevel2_flg"
  Bus Creator/1 -> Bus Selector6/1, Bus Selector5/1, Bus Selector4/1, Bus Selector3/1, Bus Selector2/1, Bus Selector18/1, Bus Selector1/1
  Bus Selector18/1 -> DAS_TFThmRnwyWarn_10ms_sys/1(GbISP_TFThmRnwyWarn_flg)  "<GbISP_TFThmRnwyWarn_flg>"
  Bus Selector18/2 -> DAS_ThmRnwyAlarmCnt_10ms_sys/1(GbISP_TFThmRnwyAlrm_flg)  "<GbISP_TFThmRnwyAlrm_flg>"
  Bus Selector18/3 -> DAS_ThmRnwyFaultCnt_10ms_sys/1(GbISP_TFThmRnwyfDet_flg)  "<GbISP_TFThmRnwyfDet_flg>"
  Bus Selector18/4 -> DAS_TPLEventWakeCnt_10ms_sys/1(GbWSM_TplWkUpPrs_flg)  "<GbWSM_TplWkUpPrs_flg>"
  Bus Selector1/1 -> DAS_HVILFailCnt_10ms_sys/1(GbISP_TFHvilLFlt_flg)  "<GbISP_TFHvilLFlt_flg>"
  Bus Selector1/2 -> DAS_HVILFailCnt_10ms_sys/2(GbISP_TFHvilSTG_flg)  "<GbISP_TFHvilSTG_flg>"
  Bus Selector1/3 -> DAS_HVILFailCnt_10ms_sys/3(GbISP_TFHvilSTV_flg)  "<GbISP_TFHvilSTV_flg>"
  Bus Selector2/1 -> DAS_IsoHVOFFChkCnt_10ms_sys/1(GbISP_TFIsoHVoffResFltLevel1_flg)  "<GbISP_TFIsoHVoffResFltLevel1_flg>"
  Bus Selector2/2 -> DAS_IsoHVOFFChkCnt_10ms_sys/2(GbISP_TFIsoHVoffResFltLevel2_flg)  "<GbISP_TFIsoHVoffResFltLevel2_flg>"
  Bus Selector3/1 -> DAS_IsoHVONChkCnt_10ms_sys/1(GbISP_TFIsoResFltLevel1_flg)  "<GbISP_TFIsoHVoffResFltLevel1_flg>"
  Bus Selector3/2 -> DAS_IsoHVONChkCnt_10ms_sys/2(GbISP_TFIsoResFltLevel2_flg)  "<GbISP_TFIsoHVoffResFltLevel2_flg>"
  Bus Selector4/1 -> DAS_IsoDCChrgChkCnt_10ms_sys/1(GbISP_TFIsoDCResFltLevel1_flg)  "<GbISP_TFIsoDCResFltLevel1_flg>"
  Bus Selector4/2 -> DAS_IsoDCChrgChkCnt_10ms_sys/2(GbISP_TFIsoDCResFltLevel2_flg)  "<GbISP_TFIsoDCResFltLevel2_flg>"
  Bus Selector5/1 -> DAS_CrashNplCnt_10ms_sys/1(GbISP_TFCANCrashFlt_flg)  "<GbISP_TFCANCrashFlt_flg>"
  Bus Selector5/2 -> DAS_CrashNplCnt_10ms_sys/2(GbISP_TFHWCrashFlt_flg)  "<GbISP_TFHWCrashFlt_flg>"
  DAS_TFThmRnwyWarn_10ms_sys/1(GcDAS_ThmRnwyWarnCnt_numb) -> GcDAS_ThmRnwyWarnCnt_numb/1
  DAS_ThmRnwyAlarmCnt_10ms_sys/1(GcDAS_ThmRnwyAlarmCnt_numb) -> GcDAS_ThmRnwyAlarmCnt_numb/1
  DAS_ThmRnwyFaultCnt_10ms_sys/1(GcDAS_ThmRnwyFaultCnt_numb) -> GcDAS_ThmRnwyFaultCnt_numb/1
  DAS_TPLEventWakeCnt_10ms_sys/1(GcDAS_TPLEventWakeCnt_numb) -> GcDAS_TPLEventWakeCnt_numb/1
  DAS_HVILFailCnt_10ms_sys/1(GcDAS_HVILFailCnt_numb) -> GcDAS_HVILFailCnt_numb/1
  DAS_IsoHVOFFChkCnt_10ms_sys/1(GcDAS_IsoHVOFFChkCnt_numb) -> GcDAS_IsoHVOFFChkCnt_numb/1
  DAS_IsoHVONChkCnt_10ms_sys/1(GcDAS_IsoHVONChkCnt_numb) -> GcDAS_IsoHVONChkCnt_numb/1
  DAS_IsoDCChrgChkCnt_10ms_sys/1(GcDAS_IsoDCChrgChkCnt_numb) -> GcDAS_IsoDCChrgChkCnt_numb/1
  DAS_CrashNplCnt_10ms_sys/1(GcDAS_CrashNplCnt_numb) -> GcDAS_CrashNplCnt_numb/1
  Bus Selector6/1 -> DAS_NVMStoreFlg_10ms_sys/1(GbISP_TFThmRnwyWarn_flg)  "<GbISP_TFThmRnwyWarn_flg>"
  Bus Selector6/2 -> DAS_NVMStoreFlg_10ms_sys/2(GbISP_TFThmRnwyAlrm_flg)  "<GbISP_TFThmRnwyAlrm_flg>"
  Bus Selector6/3 -> DAS_NVMStoreFlg_10ms_sys/3(GbISP_TFThmRnwyfDet_flg)  "<GbISP_TFThmRnwyfDet_flg>"
  Bus Selector6/4 -> DAS_NVMStoreFlg_10ms_sys/4(GbWSM_TplWkUpPrs_flg)  "<GbWSM_TplWkUpPrs_flg>"
  Bus Selector6/5 -> DAS_NVMStoreFlg_10ms_sys/5(GbISP_TFHvilLFlt_flg)  "<GbISP_TFHvilLFlt_flg>"
  Bus Selector6/6 -> DAS_NVMStoreFlg_10ms_sys/6(GbISP_TFHvilSTG_flg)  "<GbISP_TFHvilSTG_flg>"
  Bus Selector6/7 -> DAS_NVMStoreFlg_10ms_sys/7(GbISP_TFHvilSTV_flg)  "<GbISP_TFHvilSTV_flg>"
  Bus Selector6/8 -> DAS_NVMStoreFlg_10ms_sys/8(GbISP_TFIsoHVoffResFltLevel1_flg)  "<GbISP_TFIsoHVoffResFltLevel1_flg>"
  Bus Selector6/9 -> DAS_NVMStoreFlg_10ms_sys/9(GbISP_TFIsoHVoffResFltLevel2_flg)  "<GbISP_TFIsoHVoffResFltLevel2_flg>"
  Bus Selector6/10 -> DAS_NVMStoreFlg_10ms_sys/10(GbISP_TFIsoResFltLevel1_flg)  "<GbISP_TFIsoResFltLevel1_flg>"
  Bus Selector6/11 -> DAS_NVMStoreFlg_10ms_sys/11(GbISP_TFIsoResFltLevel2_flg)  "<GbISP_TFIsoResFltLevel2_flg>"
  Bus Selector6/12 -> DAS_NVMStoreFlg_10ms_sys/12(GbISP_TFIsoDCResFltLevel1_flg)  "<GbISP_TFIsoDCResFltLevel1_flg>"
  Bus Selector6/13 -> DAS_NVMStoreFlg_10ms_sys/13(GbISP_TFIsoDCResFltLevel2_flg)  "<GbISP_TFIsoDCResFltLevel2_flg>"
  Bus Selector6/14 -> DAS_NVMStoreFlg_10ms_sys/14(GbISP_TFCANCrashFlt_flg)  "<GbISP_TFCANCrashFlt_flg>"
  Bus Selector6/15 -> DAS_NVMStoreFlg_10ms_sys/15(GbISP_TFHWCrashFlt_flg)  "<GbISP_TFHWCrashFlt_flg>"
  DAS_NVMStoreFlg_10ms_sys/1(GbDAS_HVSafetyNVMStore_flg) -> GbDAS_HVSafetyNVMStore_flg/1

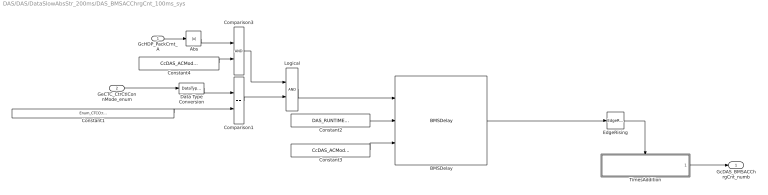
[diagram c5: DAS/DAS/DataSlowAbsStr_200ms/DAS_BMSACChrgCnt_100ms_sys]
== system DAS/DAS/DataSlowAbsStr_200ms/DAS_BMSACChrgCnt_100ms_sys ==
  GcHDP_PackCrnt_A : Inport
  GeCTC_CtrCtlConnMode_enum : Inport  Port=2
  Abs : Abs
  BMSDelay : AIWAYS_Powertrain_BMS_lib/Debounce & Delay/BMSDelay
  Comparison1 : RelationalOperator  Operator===  OutDataTypeStr=boolean
  Comparison3 : RelationalOperator  OutDataTypeStr=boolean
  Constant1 : Constant  Value=Enum_CTCCtrCtlConnMode.Enum_CTCCtrCtlConnMode_ACChrg
  Constant2 : Constant  Value=DAS_RUNTIME100_MS  OutDataTypeStr=single
  Constant3 : Constant  Value=CcDAS_ACModeCurtTiLim_ms  OutDataTypeStr=single
  Constant4 : Constant  Value=CcDAS_ACModeCurtLim_A  OutDataTypeStr=single
  Data Type Conversion : DataTypeConversion
  EdgeRising : AIWAYS_Powertrain_BMS_lib/Logical Operators/EdgeRising
  Logical : Logic  OutDataTypeStr=boolean
  TimesAddition : Subsystem  TreatAsAtomicUnit=on
  GcDAS_BMSACChrgCnt_numb : Outport
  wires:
  GcHDP_PackCrnt_A/1 -> Abs/1
  EdgeRising/1 -> TimesAddition/Enable
  TimesAddition/1(GcDAS_BMSACChrgCnt_numb) -> GcDAS_BMSACChrgCnt_numb/1
  Comparison3/1 -> Logical/1
  Constant4/1 -> Comparison3/2
  Abs/1 -> Comparison3/1
  Comparison1/1 -> Logical/2
  Logical/1 -> BMSDelay/1
  Constant2/1 -> BMSDelay/2
  Constant3/1 -> BMSDelay/3
  BMSDelay/1 -> EdgeRising/1
  GeCTC_CtrCtlConnMode_enum/1 -> Data Type Conversion/1
  Constant1/1 -> Comparison1/2
  Data Type Conversion/1 -> Comparison1/1

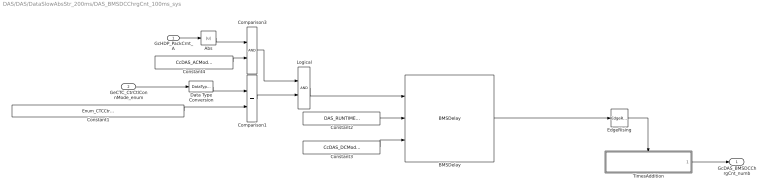
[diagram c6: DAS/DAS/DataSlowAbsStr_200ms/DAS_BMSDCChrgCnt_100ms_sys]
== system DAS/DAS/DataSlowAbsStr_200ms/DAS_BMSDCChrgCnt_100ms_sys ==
  GcHDP_PackCrnt_A : Inport
  GeCTC_CtrCtlConnMode_enum : Inport  Port=2
  Abs : Abs
  BMSDelay : AIWAYS_Powertrain_BMS_lib/Debounce & Delay/BMSDelay
  Comparison1 : RelationalOperator  Operator===  OutDataTypeStr=boolean
  Comparison3 : RelationalOperator  OutDataTypeStr=boolean
  Constant1 : Constant  Value=Enum_CTCCtrCtlConnMode.Enum_CTCCtrCtlConnMode_DCChrg
  Constant2 : Constant  Value=DAS_RUNTIME100_MS  OutDataTypeStr=single
  Constant3 : Constant  Value=CcDAS_DCModeCurtTiLim_ms  OutDataTypeStr=single
  Constant4 : Constant  Value=CcDAS_ACModeCurtLim_A  OutDataTypeStr=single
  Data Type Conversion : DataTypeConversion
  EdgeRising : AIWAYS_Powertrain_BMS_lib/Logical Operators/EdgeRising
  Logical : Logic  OutDataTypeStr=boolean
  TimesAddition : Subsystem  TreatAsAtomicUnit=on
  GcDAS_BMSDCChrgCnt_numb : Outport
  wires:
  GcHDP_PackCrnt_A/1 -> Abs/1
  EdgeRising/1 -> TimesAddition/Enable
  TimesAddition/1(GcDAS_BMSDCChrgCnt_numb) -> GcDAS_BMSDCChrgCnt_numb/1
  Comparison3/1 -> Logical/1
  Constant4/1 -> Comparison3/2
  Abs/1 -> Comparison3/1
  Comparison1/1 -> Logical/2
  Logical/1 -> BMSDelay/1
  Constant2/1 -> BMSDelay/2
  Constant3/1 -> BMSDelay/3
  BMSDelay/1 -> EdgeRising/1
  GeCTC_CtrCtlConnMode_enum/1 -> Data Type Conversion/1
  Constant1/1 -> Comparison1/2
  Data Type Conversion/1 -> Comparison1/1

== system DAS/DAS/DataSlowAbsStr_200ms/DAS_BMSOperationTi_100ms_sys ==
  Constant1 : Constant  Value=boolean(1)
  Constant2 : Constant  Value=CcDAS_BMSOperationConfirmTi_ms
  Constant3 : Constant  Value=DAS_RUNTIME100_MS
  Data Type Conversion : DataTypeConversion  OutDataTypeStr=uint16
  OperationTimeCalc : Subsystem
  Turn On Delay Time : AIWAYS_Powertrain_BMS_lib/Delay Blocks/Turn On Delay Time
  GcDAS_BMSOperationTi_min : Outport
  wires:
  OperationTimeCalc/1(GcDAS_BMSOperationTi_min) -> GcDAS_BMSOperationTi_min/1
  Constant1/1 -> Turn On Delay Time/2
  Constant3/1 -> Data Type Conversion/1
  Constant2/1 -> Turn On Delay Time/1
  Turn On Delay Time/1 -> OperationTimeCalc/Enable
  Data Type Conversion/1 -> Turn On Delay Time/3

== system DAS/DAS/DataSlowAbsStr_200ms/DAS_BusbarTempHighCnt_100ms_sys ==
  GbISP_TFBusbarTempHiFltLv3_flg : Inport
  EdgeRising : AIWAYS_Powertrain_BMS_lib/Logical Operators/EdgeRising
  TimesAddition : Subsystem  TreatAsAtomicUnit=on
  GcDAS_BusbarTempHighCnt_numb : Outport
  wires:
  GbISP_TFBusbarTempHiFltLv3_flg/1 -> EdgeRising/1
  EdgeRising/1 -> TimesAddition/Enable
  TimesAddition/1(GcDAS_BusbarTempHighCnt_numb) -> GcDAS_BusbarTempHighCnt_numb/1

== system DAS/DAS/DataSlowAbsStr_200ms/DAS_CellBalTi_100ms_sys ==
  GaCBC_CellBalCtlCmd_flg : Inport
  Logical1 : Logic  Operator=OR  Inputs=1  OutDataTypeStr=boolean
  OperationTimeCalc : Subsystem
  GcDAS_CellBalTi_min : Outport
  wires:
  GaCBC_CellBalCtlCmd_flg/1 -> Logical1/1
  OperationTimeCalc/1(GcDAS_CellBalTi_min) -> GcDAS_CellBalTi_min/1
  Logical1/1 -> OperationTimeCalc/Enable

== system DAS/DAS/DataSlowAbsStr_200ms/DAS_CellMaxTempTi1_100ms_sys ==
  GcCDP_MaxCellTemp_C : Inport
  GbCDP_AllCellTempVld_flg : Inport  Port=2
  GcCDP_MinCellTemp_C : Inport  Port=3
  Comparison1 : RelationalOperator  OutDataTypeStr=boolean
  Comparison2 : RelationalOperator  Operator=<  OutDataTypeStr=boolean
  Comparison3 : RelationalOperator  Operator=>  OutDataTypeStr=boolean
  Constant1 : Constant  Value=CcDAS_CellMaxTempLim2_C
  Constant7 : Constant  Value=CcDAS_CellMaxTempLim1_C
  Logical : Logic  Inputs=3  OutDataTypeStr=boolean
  Logical1 : Logic  OutDataTypeStr=boolean
  OperationTimeCalc : Subsystem
  GcDAS_CellMaxTempTi1_min : Outport
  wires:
  GcCDP_MaxCellTemp_C/1 -> Comparison1/2, Comparison3/1
  Constant7/1 -> Comparison2/1, Comparison3/2
  Comparison3/1 -> Logical1/2
  GbCDP_AllCellTempVld_flg/1 -> Logical/3
  Logical/1 -> OperationTimeCalc/Enable
  OperationTimeCalc/1(GcDAS_CellMaxTempTi1_min) -> GcDAS_CellMaxTempTi1_min/1
  Constant1/1 -> Comparison1/1
  Comparison1/1 -> Logical1/1
  Logical1/1 -> Logical/1
  Comparison2/1 -> Logical/2
  GcCDP_MinCellTemp_C/1 -> Comparison2/2

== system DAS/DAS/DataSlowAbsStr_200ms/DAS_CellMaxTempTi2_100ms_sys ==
  GcCDP_MaxCellTemp_C : Inport
  GbCDP_AllCellTempVld_flg : Inport  Port=2
  Comparison1 : RelationalOperator  OutDataTypeStr=boolean
  Comparison3 : RelationalOperator  Operator=>  OutDataTypeStr=boolean
  Constant1 : Constant  Value=CcDAS_CellMaxTempLim3_C
  Constant7 : Constant  Value=CcDAS_CellMaxTempLim2_C
  Logical : Logic  OutDataTypeStr=boolean
  Logical1 : Logic  OutDataTypeStr=boolean
  OperationTimeCalc : Subsystem
  GcDAS_CellMaxTempTi2_min : Outport
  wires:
  GcCDP_MaxCellTemp_C/1 -> Comparison1/2, Comparison3/1
  Constant7/1 -> Comparison3/2
  Comparison3/1 -> Logical1/2
  GbCDP_AllCellTempVld_flg/1 -> Logical/2
  Logical/1 -> OperationTimeCalc/Enable
  OperationTimeCalc/1(GcDAS_CellMaxTempTi2_min) -> GcDAS_CellMaxTempTi2_min/1
  Constant1/1 -> Comparison1/1
  Comparison1/1 -> Logical1/1
  Logical1/1 -> Logical/1

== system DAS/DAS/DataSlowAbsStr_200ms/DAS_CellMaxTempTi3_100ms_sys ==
  GcCDP_MaxCellTemp_C : Inport
  GbCDP_AllCellTempVld_flg : Inport  Port=2
  Comparison1 : RelationalOperator  OutDataTypeStr=boolean
  Comparison3 : RelationalOperator  Operator=>  OutDataTypeStr=boolean
  Constant1 : Constant  Value=CcDAS_CellMaxTempLim4_C
  Constant7 : Constant  Value=CcDAS_CellMaxTempLim3_C
  Logical : Logic  OutDataTypeStr=boolean
  Logical1 : Logic  OutDataTypeStr=boolean
  OperationTimeCalc : Subsystem
  GcDAS_CellMaxTempTi3_min : Outport
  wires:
  GcCDP_MaxCellTemp_C/1 -> Comparison1/2, Comparison3/1
  Constant7/1 -> Comparison3/2
  Comparison3/1 -> Logical1/2
  GbCDP_AllCellTempVld_flg/1 -> Logical/2
  Logical/1 -> OperationTimeCalc/Enable
  OperationTimeCalc/1(GcDAS_CellMaxTempTi3_min) -> GcDAS_CellMaxTempTi3_min/1
  Constant1/1 -> Comparison1/1
  Comparison1/1 -> Logical1/1
  Logical1/1 -> Logical/1

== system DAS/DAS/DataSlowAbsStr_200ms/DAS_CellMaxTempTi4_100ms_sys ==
  GcCDP_MaxCellTemp_C : Inport
  GbCDP_AllCellTempVld_flg : Inport  Port=2
  Comparison3 : RelationalOperator  Operator=>  OutDataTypeStr=boolean
  Constant7 : Constant  Value=CcDAS_CellMaxTempLim4_C
  Logical : Logic  OutDataTypeStr=boolean
  OperationTimeCalc : Subsystem
  GcDAS_CellMaxTempTi4_min : Outport
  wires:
  GcCDP_MaxCellTemp_C/1 -> Comparison3/1
  Constant7/1 -> Comparison3/2
  Comparison3/1 -> Logical/1
  GbCDP_AllCellTempVld_flg/1 -> Logical/2
  Logical/1 -> OperationTimeCalc/Enable
  OperationTimeCalc/1(GcDAS_CellMaxTempTi4_min) -> GcDAS_CellMaxTempTi4_min/1

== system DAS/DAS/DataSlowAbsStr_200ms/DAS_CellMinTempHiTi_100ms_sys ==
  GcCDP_MinCellTemp_C : Inport
  GbCDP_AllCellTempVld_flg : Inport  Port=2
  Comparison1 : RelationalOperator  OutDataTypeStr=boolean
  Comparison3 : RelationalOperator  Operator=>  OutDataTypeStr=boolean
  Constant1 : Constant  Value=CcDAS_CellMinTempHiLim_C
  Constant7 : Constant  Value=CcDAS_CellMinTempMidLim_C
  Logical : Logic  OutDataTypeStr=boolean
  Logical1 : Logic  OutDataTypeStr=boolean
  OperationTimeCalc : Subsystem
  GcDAS_CellMinTempHiTi_min : Outport
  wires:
  GcCDP_MinCellTemp_C/1 -> Comparison1/2, Comparison3/1
  Constant7/1 -> Comparison3/2
  Comparison3/1 -> Logical1/2
  GbCDP_AllCellTempVld_flg/1 -> Logical/2
  Logical/1 -> OperationTimeCalc/Enable
  OperationTimeCalc/1(GcDAS_CellMinTempHiTi_min) -> GcDAS_CellMinTempHiTi_min/1
  Constant1/1 -> Comparison1/1
  Comparison1/1 -> Logical1/1
  Logical1/1 -> Logical/1

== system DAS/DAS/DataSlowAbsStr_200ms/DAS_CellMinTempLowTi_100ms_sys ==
  GcCDP_MinCellTemp_C : Inport
  GbCDP_AllCellTempVld_flg : Inport  Port=2
  Comparison3 : RelationalOperator  Operator=<=  OutDataTypeStr=boolean
  Constant7 : Constant  Value=CcDAS_CellMinTempLowLim_C
  Logical : Logic  OutDataTypeStr=boolean
  OperationTimeCalc : Subsystem
  GcDAS_CellMinTempLowTi_min : Outport
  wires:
  GcCDP_MinCellTemp_C/1 -> Comparison3/1
  Constant7/1 -> Comparison3/2
  Comparison3/1 -> Logical/1
  GbCDP_AllCellTempVld_flg/1 -> Logical/2
  Logical/1 -> OperationTimeCalc/Enable
  OperationTimeCalc/1(GcDAS_CellMinTempLowTi_min) -> GcDAS_CellMinTempLowTi_min/1

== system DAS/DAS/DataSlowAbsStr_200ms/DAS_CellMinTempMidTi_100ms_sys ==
  GcCDP_MinCellTemp_C : Inport
  GbCDP_AllCellTempVld_flg : Inport  Port=2
  Comparison1 : RelationalOperator  OutDataTypeStr=boolean
  Comparison3 : RelationalOperator  Operator=>  OutDataTypeStr=boolean
  Constant1 : Constant  Value=CcDAS_CellMinTempMidLim_C
  Constant7 : Constant  Value=CcDAS_CellMinTempLowLim_C
  Logical : Logic  OutDataTypeStr=boolean
  Logical1 : Logic  OutDataTypeStr=boolean
  OperationTimeCalc : Subsystem
  GcDAS_CellMinTempMidTi_min : Outport
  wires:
  Logical1/1 -> Logical/1
  Comparison1/1 -> Logical1/1
  Constant1/1 -> Comparison1/1
  OperationTimeCalc/1(GcDAS_CellMinTempMidTi_min) -> GcDAS_CellMinTempMidTi_min/1
  Logical/1 -> OperationTimeCalc/Enable
  GbCDP_AllCellTempVld_flg/1 -> Logical/2
  Comparison3/1 -> Logical1/2
  Constant7/1 -> Comparison3/2
  GcCDP_MinCellTemp_C/1 -> Comparison3/1, Comparison1/2

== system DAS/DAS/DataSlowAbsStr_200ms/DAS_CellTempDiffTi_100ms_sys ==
  GcCDP_MaxCellTemp_C : Inport
  GbCDP_AllCellTempVld_flg : Inport  Port=2
  GcCDP_MinCellTemp_C : Inport  Port=3
  Comparison1 : RelationalOperator  Operator=>  OutDataTypeStr=boolean
  Constant1 : Constant  Value=CcDAS_CellTempDiffLim_C
  Logical : Logic  OutDataTypeStr=boolean
  OperationTimeCalc : Subsystem
  Sum1 : Sum  Inputs=+-  OutDataTypeStr=Inherit: Inherit via back propagation  RndMeth=Zero
  GcDAS_CellTempDiffLimTi_min : Outport
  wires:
  GcCDP_MaxCellTemp_C/1 -> Sum1/1
  GbCDP_AllCellTempVld_flg/1 -> Logical/2
  Logical/1 -> OperationTimeCalc/Enable
  OperationTimeCalc/1(GcDAS_CellTempDiffLimTi_min) -> GcDAS_CellTempDiffLimTi_min/1
  Constant1/1 -> Comparison1/2
  Comparison1/1 -> Logical/1
  GcCDP_MinCellTemp_C/1 -> Sum1/2
  Sum1/1 -> Comparison1/1

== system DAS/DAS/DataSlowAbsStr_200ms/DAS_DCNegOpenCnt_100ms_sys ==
  GbISP_TFDCNegOpenFlt_flg : Inport
  EdgeRising : AIWAYS_Powertrain_BMS_lib/Logical Operators/EdgeRising
  TimesAddition : Subsystem  TreatAsAtomicUnit=on
  GcDAS_DCNegOpenCnt_numb : Outport
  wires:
  GbISP_TFDCNegOpenFlt_flg/1 -> EdgeRising/1
  EdgeRising/1 -> TimesAddition/Enable
  TimesAddition/1(GcDAS_DCNegOpenCnt_numb) -> GcDAS_DCNegOpenCnt_numb/1

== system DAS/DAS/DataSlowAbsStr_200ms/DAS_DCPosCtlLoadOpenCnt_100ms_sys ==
  GcISP_ShutDownDCPosChrgCtlLoadOpen_flg : Inport
  EdgeRising : AIWAYS_Powertrain_BMS_lib/Logical Operators/EdgeRising
  TimesAddition : Subsystem  TreatAsAtomicUnit=on
  GcDAS_DCPosCtlLoadOpenCnt_numb : Outport
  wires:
  GcISP_ShutDownDCPosChrgCtlLoadOpen_flg/1 -> EdgeRising/1
  EdgeRising/1 -> TimesAddition/Enable
  TimesAddition/1(GcDAS_DCPosCtlLoadOpenCnt_numb) -> GcDAS_DCPosCtlLoadOpenCnt_numb/1

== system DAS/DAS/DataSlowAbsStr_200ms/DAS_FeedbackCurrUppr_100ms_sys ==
  GbISP_TFFeedbackPwrFltLevel3_flg : Inport
  EdgeRising : AIWAYS_Powertrain_BMS_lib/Logical Operators/EdgeRising
  TimesAddition : Subsystem  TreatAsAtomicUnit=on
  GcDAS_FeedbackCurrUpprLimCnt_numb : Outport
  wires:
  GbISP_TFFeedbackPwrFltLevel3_flg/1 -> EdgeRising/1
  EdgeRising/1 -> TimesAddition/Enable
  TimesAddition/1(GcDAS_FeedbackCurrUpprLimCnt_numb) -> GcDAS_FeedbackCurrUpprLimCnt_numb/1

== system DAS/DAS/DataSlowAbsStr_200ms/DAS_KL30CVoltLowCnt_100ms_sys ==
  GbISP_TFKL30CStTooLow_flg : Inport
  EdgeRising : AIWAYS_Powertrain_BMS_lib/Logical Operators/EdgeRising
  Logical1 : Logic  Operator=OR  OutDataTypeStr=boolean
  TimesAddition : Subsystem  TreatAsAtomicUnit=on
  Unit Delay21 : UnitDelay  SampleTime=-1  StateName=StateName
  GcDAS_KL30CVoltLowCnt_numb : Outport
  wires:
  EdgeRising/1 -> TimesAddition/Enable
  TimesAddition/1(GcDAS_KL30CVoltLowCnt_numb) -> GcDAS_KL30CVoltLowCnt_numb/1
  Logical1/1 -> Unit Delay21/1, EdgeRising/1
  Unit Delay21/1 -> Logical1/1
  GbISP_TFKL30CStTooLow_flg/1 -> Logical1/2

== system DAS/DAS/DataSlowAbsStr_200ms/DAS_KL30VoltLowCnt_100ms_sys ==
  GbISP_TFBMUSpyStTooLow_flg : Inport
  EdgeRising : AIWAYS_Powertrain_BMS_lib/Logical Operators/EdgeRising
  Logical1 : Logic  Operator=OR  OutDataTypeStr=boolean
  TimesAddition : Subsystem  TreatAsAtomicUnit=on
  Unit Delay21 : UnitDelay  SampleTime=-1  StateName=StateName
  GcDAS_KL30VoltLowCnt_numb : Outport
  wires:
  EdgeRising/1 -> TimesAddition/Enable
  TimesAddition/1(GcDAS_KL30VoltLowCnt_numb) -> GcDAS_KL30VoltLowCnt_numb/1
  Logical1/1 -> Unit Delay21/1, EdgeRising/1
  Unit Delay21/1 -> Logical1/1
  GbISP_TFBMUSpyStTooLow_flg/1 -> Logical1/2

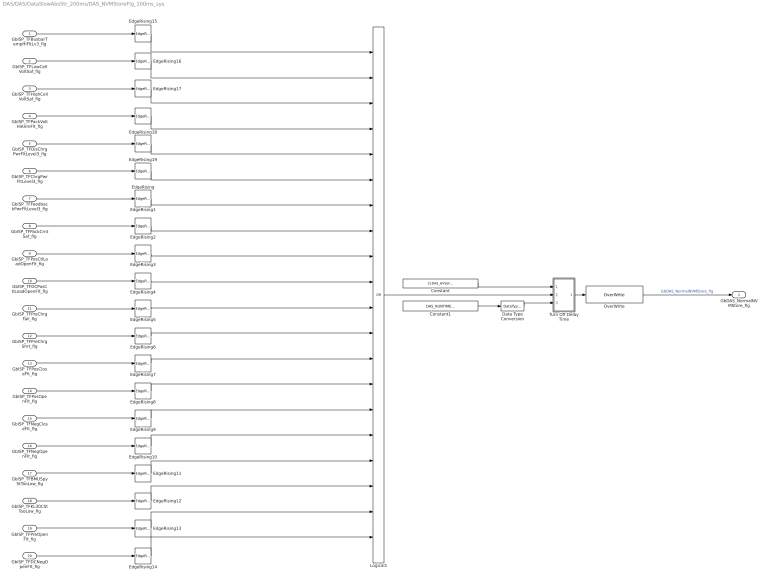
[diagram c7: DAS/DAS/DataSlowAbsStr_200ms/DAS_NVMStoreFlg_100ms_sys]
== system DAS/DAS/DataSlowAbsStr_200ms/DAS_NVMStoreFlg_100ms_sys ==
  GbISP_TFBusbarTempHiFltLv3_flg : Inport
  GbISP_TFLowCellVoltSaf_flg : Inport  Port=2
  GbISP_TFHighCellVoltSaf_flg : Inport  Port=3
  GbISP_TFPackVoltHiAlrmFlt_flg : Inport  Port=4
  GbISP_TFDisChrgPwrFltLevel3_flg : Inport  Port=5
  GbISP_TFChrgPwrFltLevel3_flg : Inport  Port=6
  GbISP_TFFeedbackPwrFltLevel3_flg : Inport  Port=7
  GbISP_TFPackCrntSaf_flg : Inport  Port=8
  GbISP_TFPosCtlLoadOpenFlt_flg : Inport  Port=9
  GbISP_TFDCPosCtlLoadOpenFlt_flg : Inport  Port=10
  GbISP_TFPreChrgFail_flg : Inport  Port=11
  GbISP_TFPreChrgShrt_flg : Inport  Port=12
  GbISP_TFPosCloseFlt_flg : Inport  Port=13
  GbISP_TFPosOpenFlt_flg : Inport  Port=14
  GbISP_TFNegCloseFlt_flg : Inport  Port=15
  GbISP_TFNegOpenFlt_flg : Inport  Port=16
  GbISP_TFBMUSpyStTooLow_flg : Inport  Port=17
  GbISP_TFKL30CStTooLow_flg : Inport  Port=18
  GbISP_TFPreOpenFlt_flg : Inport  Port=19
  GbISP_TFDCNegOpenFlt_flg : Inport  Port=20
  Constant : Constant  Value=CcDAS_HVSafetyNVMStoreTi_ms
  Constant1 : Constant  Value=DAS_RUNTIME100_MS
  Data Type Conversion : DataTypeConversion  OutDataTypeStr=uint16
  EdgeRising{,1..19} (20 alike) : AIWAYS_Powertrain_BMS_lib/Logical Operators/EdgeRising
  Logical1 : Logic  Operator=OR  Inputs=20  OutDataTypeStr=boolean
  OverWrite : AIWAYS_Powertrain_BMS_lib/Signals/OverWrite  OverWrite_Value=CbDAS_NormalNVMStoreOvr_flg  OverWrite_flag=CbDAS_NormalNVMStoreOvrSwt_flg
  Turn Off Delay Time : Subsystem  TreatAsAtomicUnit=on  mask(TurnOffDelayTime){}
      mask help: The falling edge of the input signal (u) is delayed by the input delay time (T). Input1= Delay Time; Input2=Signal (u); Input3=Activation Rate.
  GbDAS_NormalNVMStore_flg : Outport
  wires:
  EdgeRising12/1 -> Logical1/18
  EdgeRising3/1 -> Logical1/9
  EdgeRising8/1 -> Logical1/14
  EdgeRising7/1 -> Logical1/13
  EdgeRising1/1 -> Logical1/7
  EdgeRising10/1 -> Logical1/16
  EdgeRising2/1 -> Logical1/8
  EdgeRising5/1 -> Logical1/11
  EdgeRising/1 -> Logical1/6
  EdgeRising11/1 -> Logical1/17
  EdgeRising9/1 -> Logical1/15
  EdgeRising14/1 -> Logical1/20
  EdgeRising13/1 -> Logical1/19
  EdgeRising6/1 -> Logical1/12
  EdgeRising4/1 -> Logical1/10
  GbISP_TFDCNegOpenFlt_flg/1 -> EdgeRising14/1
  GbISP_TFPreOpenFlt_flg/1 -> EdgeRising13/1
  GbISP_TFKL30CStTooLow_flg/1 -> EdgeRising12/1
  GbISP_TFBMUSpyStTooLow_flg/1 -> EdgeRising11/1
  GbISP_TFNegOpenFlt_flg/1 -> EdgeRising10/1
  GbISP_TFNegCloseFlt_flg/1 -> EdgeRising9/1
  GbISP_TFPosOpenFlt_flg/1 -> EdgeRising8/1
  GbISP_TFPosCloseFlt_flg/1 -> EdgeRising7/1
  GbISP_TFPreChrgShrt_flg/1 -> EdgeRising6/1
  GbISP_TFPreChrgFail_flg/1 -> EdgeRising5/1
  GbISP_TFDCPosCtlLoadOpenFlt_flg/1 -> EdgeRising4/1
  GbISP_TFPosCtlLoadOpenFlt_flg/1 -> EdgeRising3/1
  GbISP_TFPackCrntSaf_flg/1 -> EdgeRising2/1
  GbISP_TFFeedbackPwrFltLevel3_flg/1 -> EdgeRising1/1
  GbISP_TFChrgPwrFltLevel3_flg/1 -> EdgeRising/1
  GbISP_TFDisChrgPwrFltLevel3_flg/1 -> EdgeRising19/1
  GbISP_TFBusbarTempHiFltLv3_flg/1 -> EdgeRising15/1
  GbISP_TFLowCellVoltSaf_flg/1 -> EdgeRising16/1
  GbISP_TFHighCellVoltSaf_flg/1 -> EdgeRising17/1
  GbISP_TFPackVoltHiAlrmFlt_flg/1 -> EdgeRising18/1
  EdgeRising15/1 -> Logical1/1
  EdgeRising16/1 -> Logical1/2
  EdgeRising17/1 -> Logical1/3
  EdgeRising18/1 -> Logical1/4
  EdgeRising19/1 -> Logical1/5
  Logical1/1 -> Turn Off Delay Time/2(u)
  Constant1/1 -> Data Type Conversion/1
  Constant/1 -> Turn Off Delay Time/1(T)
  Turn Off Delay Time/1(y) -> OverWrite/1
  OverWrite/1 -> GbDAS_NormalNVMStore_flg/1  "GbDAS_NormalNVMStore_flg"
  Data Type Conversion/1 -> Turn Off Delay Time/3(dT)
